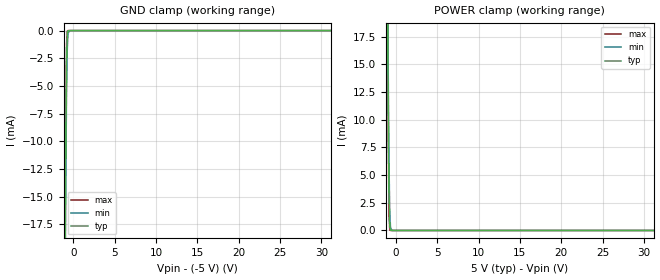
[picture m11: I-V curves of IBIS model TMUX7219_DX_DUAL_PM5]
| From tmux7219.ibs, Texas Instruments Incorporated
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[Model]   TMUX7219_DX_DUAL_PM5
Model_type   Terminator
|   typ   min   max
C_comp   60pF   60pF   60pF
[Voltage Range]   30   27   33
[Temperature Range]   27   130   -40
[Power Clamp Reference]   5   5   5
[GND Clamp Reference]   -5   -5   -5
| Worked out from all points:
|   GND clamp passes 1 mA (typ) near -0.77 V on its own axis
|   POWER clamp passes 1 mA (typ) near -0.77 V on its own axis
[GND Clamp]
|   Voltage   I(typ)   I(min)   I(max)
-30V      -4.646A    -4.714A    -4.649A
-1.02V    -22.01mA   -24.41mA   -19.81mA
-930mV    -11.04mA   -13.89mA   -8.565mA
-840mV    -3.269mA   -5.934mA   -1.414mA
-750mV    -384.6uA   -1.761mA   -36.11uA
-660mV    -13.98uA   -270.8uA   -471.2nA
-480mV    -8.39uA    -1.291uA   0A
-210mV    0A         0A         0A
60V       0A         0A         0A
[POWER Clamp]
|   Voltage   I(typ)   I(min)   I(max)
-30V      4.646A     4.714A     4.649A
-1.02V    22.01mA    24.41mA    19.81mA
-930mV    11.04mA    13.89mA    8.565mA
-840mV    3.269mA    5.934mA    1.414mA
-750mV    384.6uA    1.761mA    36.11uA
-660mV    13.98uA    270.8uA    471.2nA
-480mV    8.39uA     1.291uA    0A
-210mV    0A         0A         0A
60V       0A         0A         0A
